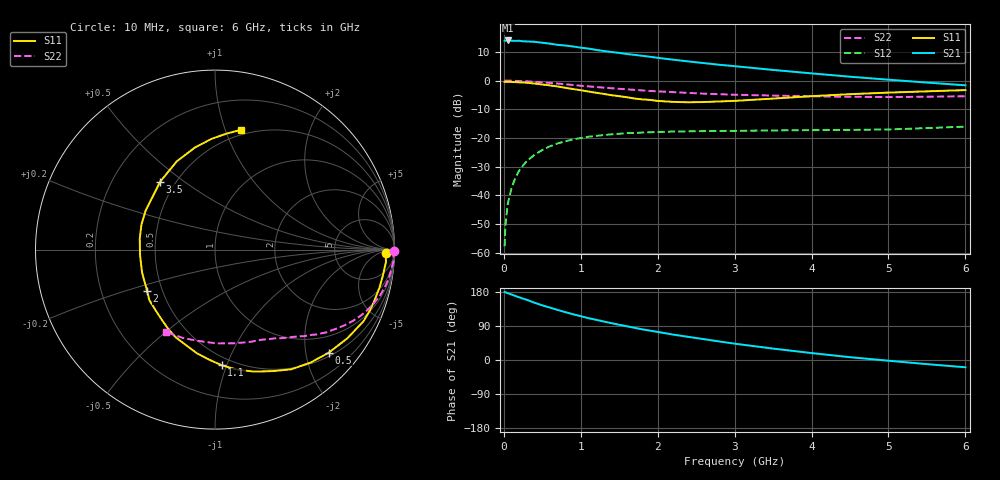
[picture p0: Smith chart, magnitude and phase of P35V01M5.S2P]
! SIEMENS Small Signal Semiconductors
! BFP181
! Si NPN RF Bipolar Junction Transistor in SOT143
! VCE = 5 V  IC = 1.5 mA
! Common Emitter S-Parameters:  March  1996
# GHz  S  MA  R  50
!  f  S11  S21  S12  S22
! GHz  MAG  ANG  MAG  ANG  MAG  ANG  MAG  ANG
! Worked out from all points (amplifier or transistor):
!   36 points, 10 MHz to 6 GHz, reference 50 ohm
!   highest |S21| = 14.0 dB at 50 MHz (marker M1)
!   |S21| within 3 dB of that: start of sweep to 1.136 GHz
!   unconditionally stable (mu >= 1): 2.789 GHz to end of sweep
!   at 250 MHz: K = 0.10, MSG = 21.6 dB, |S12| = -29.6 dB
!   at 1.4 GHz: K = 0.57, MSG = 14.3 dB, |S12| = -18.7 dB
!   at 6 GHz: K = 1.21, MAG = 4.5 dB, |S12| = -16.0 dB
!   S11 on the Smith chart (normalised r, x): 10 MHz: 36, -13; 500 MHz: 0.58, -2.47; 1.1 GHz: 0.43, -0.96; 2 GHz: 0.41, -0.24; 3.5 GHz: 0.41, +0.41; 6 GHz: 0.45, +1.14
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0.01  0.9524 -1.0  4.986 179.4  0.0013 84.8  0.997 -0.3
0.02  0.9517 -1.7  4.948 179.0  0.0029 79.7  0.9998 -0.8
0.05  0.955 -4.1  5.015 176.3  0.007 90.5  0.9956 -2.0
0.1  0.9466 -8.7  4.954 172.8  0.0134 82.7  0.9959 -4.0
0.2  0.9334 -17.3  4.951 165.3  0.027 79.6  0.9849 -7.9
0.4  0.888 -33.8  4.75 151.0  0.0511 68.8  0.9553 -15.4
0.5  0.8551 -42.2  4.576 144.2  0.0618 63.4  0.9334 -18.8
0.6  0.8248 -49.7  4.412 138.2  0.0717 59.1  0.9109 -22.0
0.8  0.749 -64.7  4.09 126.2  0.0876 51.3  0.8644 -27.4
0.9  0.7134 -72.3  3.937 120.7  0.0947 47.3  0.8386 -30.0
1.1  0.6455 -86.7  3.618 110.4  0.1052 41.0  0.7933 -34.4
1.3  0.5858 -100.0  3.285 101.5  0.1125 35.6  0.7548 -38.2
1.5  0.5355 -114.2  3.044 92.9  0.1185 31.1  0.7196 -41.3
1.8  0.4706 -135.7  2.707 80.9  0.1242 25.9  0.6743 -45.7
2  0.4428 -148.7  2.498 74.1  0.1272 22.9  0.6506 -48.4
2.2  0.4261 -162.4  2.319 67.1  0.1295 20.1  0.6308 -51.2
2.8  0.433 161.2  1.891 48.9  0.1325 14.6  0.5807 -59.3
3.5  0.4863 128.9  1.536 30.1  0.1355 10.5  0.5489 -69.8
4  0.536 113.4  1.338 18.3  0.137 8.6  0.5321 -78.9
4.5  0.5802 101.0  1.17 7.4  0.1384 7.4  0.5228 -88.9
5.5  0.6504 84.1  0.925 -10.9  0.1488 7.6  0.5238 -109.8
6  0.6837 77.6  0.829 -19.2  0.1578 6.7  0.5343 -120.6
